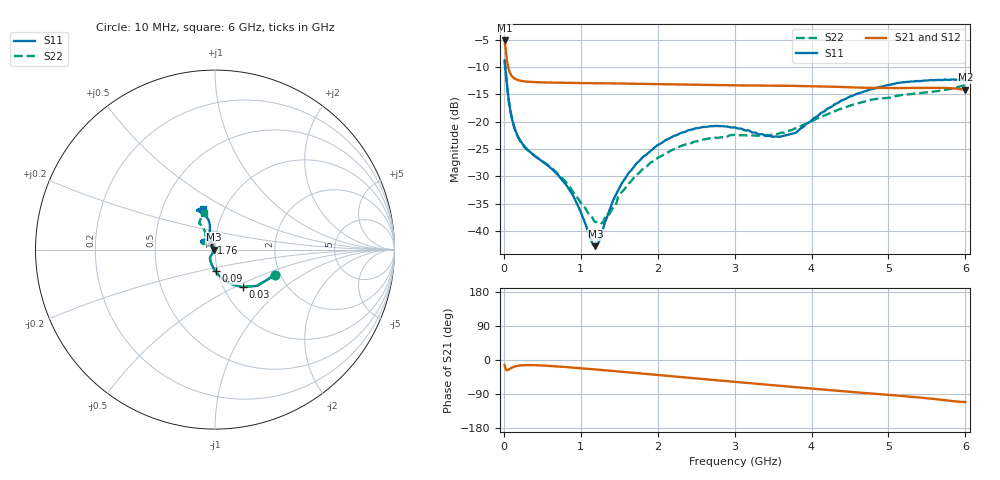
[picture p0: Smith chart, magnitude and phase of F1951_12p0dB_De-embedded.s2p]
! Integrated Device Technology
! Corporate Headquarters
! 6024 Silver Creek Valley Road
! San Jose, CA 95138  USA
! Phone:  1-408-284-8200
! Toll Free:  1-800-223-1366
! Webpage:  http://www.idt.com/
! Timing and RF Division
! 515 Groton Road, Suite 102
! Westford, MA 01886-6024
! Device:  F1951
! Description: 6-bit 0.5 dB Digital Step Attenuator
! Frequency:  100.0 -  4000.00 MHz
! Package:  4x4 mm Thin QFN Plastic Package: 24 pin
! Ports:  2 RF, 6 DC
!  Pin  1  = NC
!  Pin  2  = RF1  =  Port 1
!  Pin  3  = GND
!  Pin  4  = NC
!  Pin  5  = Serial Data Out (SDO)
!  Pin  6  = NC
!  Pin  7  = Reset Bar ( RSTb)
!  Pin  8  = Clock (CLK)
!  Pin  9  = Chip Select Bar (CSb)
!  Pin 10  = NC
!  Pin 11  = Serial Data In (SDI)
!  Pin 12  = NC
!  Pin 13  = NC
!  Pin 14  = VDD
!  Pin 15  = NC
!  Pin 16  = GND
!  Pin 17  = RF2  =  Port 2
!  Pin 18  = NC
!  Pin 19  = GND
!  Pin 20  = GND
!  Pin 21  = GND
!  Pin 22  = GND
!  Pin 23  = GND
!  Pin 24  = GND
! State:  24
! Atten State:  12.0 dB
! Voltage:  +3.30 Volts
! Current:  0.472 mA
! Data:  The device was measured on a F195X evaluation board which has
!  individual transmission lines to the RF pins.  Data was collected
!  de-embedded using a Automatic Fixture Removal [AFR] (Keysight Technologies).
!  The reference plane is the edge of the package pin.
! Misc:  Lot Code  1225BCA
!  Action Tracker AT0399
! Date Measured:  2018-09-13
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# GHz S dB R 50
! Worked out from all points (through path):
!   600 points, 10 MHz to 6 GHz, reference 50 ohm
!   highest |S21| = -5.14 dB at 10 MHz (marker M1); lowest = -14.2 dB at 6 GHz (marker M2)
!   group delay of S21, straight-line fit = 47.4 ps
!   lowest |S11| = -42.8 dB at 1.19 GHz (marker M3), VSWR 1.01, Z = 49.3 + j0.0515 ohm
!   |S11| at or under -10 dB: 18.8 MHz to end of sweep
!   |S22| runs from -38.6 to -8.8 dB; largest |S21 - S12| = 0.00043
!   S11 on the Smith chart (normalised r, x): 10 MHz: 1.88, -0.61; 30 MHz: 1.23, -0.55; 90 MHz: 0.98, -0.24; 1.76 GHz: 0.96, +0.07; 6 GHz: 0.79, +0.38
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0.01  -8.78 -22.8  -5.14 -13.4  -5.14 -13.4  -8.83 -22.9
0.03  -11.72 -53.6  -7.64 -25.9  -7.64 -26.0  -11.77 -53.7
0.06  -15.67 -76.2  -10.22 -25.6  -10.22 -25.6  -15.75 -76.4
0.09  -18.39 -88.6  -11.36 -21.7  -11.37 -21.7  -18.46 -88.9
0.16  -21.98 -105.5  -12.28 -16.3  -12.28 -16.3  -22.08 -105.5
0.26  -24.40 -117.0  -12.62 -13.7  -12.62 -13.7  -24.55 -117.5
0.72  -30.03 -123.1  -12.88 -17.3  -12.88 -17.3  -29.80 -127.5
1.01  -36.93 -129.2  -12.95 -21.9  -12.96 -21.9  -35.04 -133.4
1.14  -41.90 -159.0  -12.97 -24.0  -12.97 -24.0  -37.34 -149.6
1.19  -42.81 175.9  -12.97 -24.9  -12.98 -24.9  -38.40 -160.3
1.29  -39.68 134.0  -12.98 -26.6  -12.99 -26.6  -38.39 173.6
1.5  -32.22 116.3  -13.03 -30.3  -13.04 -30.3  -33.39 143.8
1.76  -27.23 119.1  -13.07 -35.1  -13.07 -35.1  -29.38 136.1
2.01  -24.22 126.6  -13.13 -39.7  -13.13 -39.7  -26.54 139.3
2.49  -21.22 141.2  -13.24 -48.4  -13.24 -48.4  -23.65 148.7
3.01  -21.10 152.2  -13.36 -57.7  -13.36 -57.6  -22.43 152.9
3.59  -22.76 131.5  -13.41 -68.0  -13.42 -68.0  -22.10 135.0
3.79  -22.08 116.4  -13.48 -71.6  -13.48 -71.6  -21.23 127.7
4.01  -19.62 106.2  -13.51 -75.5  -13.51 -75.5  -19.90 121.5
4.49  -15.47 102.5  -13.71 -83.8  -13.71 -83.8  -17.12 118.9
5.01  -13.29 110.5  -13.87 -92.0  -13.87 -92.0  -15.63 120.8
6  -12.48 106.4  -14.16 -110.9  -14.16 -110.9  -13.31 107.1
